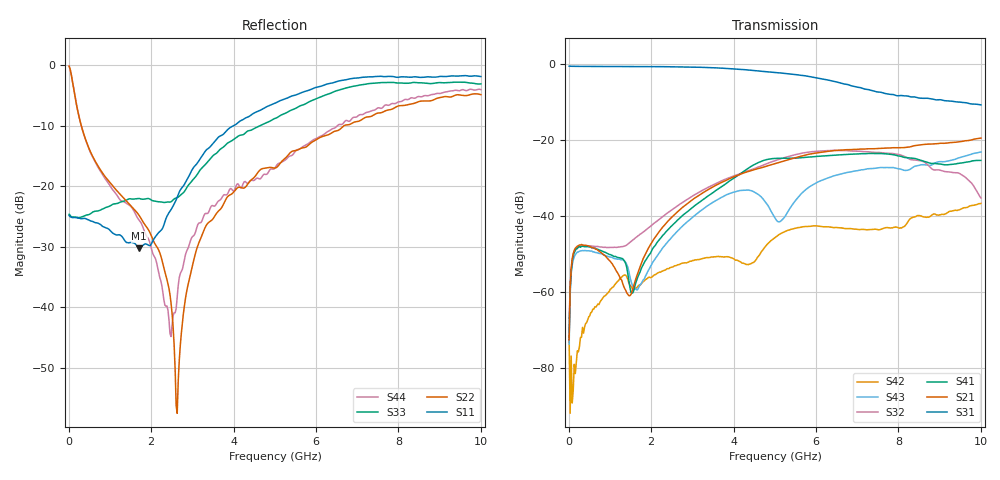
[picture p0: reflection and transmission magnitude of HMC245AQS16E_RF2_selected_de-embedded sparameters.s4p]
! Device:	HMC245AQS16E
! Description:	GaAs MMIC SP3T Non-Reflective Switch
! Package:	LP3E - 16 pin 3x3mm QFN plastic package
! Frequency:	DC -  3.5 GHz
! Ports:
! RFC = Port 1
! RF1 = Port 2
! RF2 = Port 3
! RF3 = Port 4
! State: RF2 Selected
! Supply Voltage:
! Vdd = 5 V
! Control Voltages:
! VA  = 5 V
! VB  = 0 V
! Data:	Data was collected using a calibrated network analyzer with AFR software.
!	Fixtures were calculated using AFR and fixturing was applied to collect
!	this Deembedded  S Parameter data of HMC245AQS16E
! Note:	Analog Devices supplies this data as a sample of measured data at the package pin
!	for this product.  Your particular data for this product may vary.
!	Data was taken at 25 degrees C.
!	Analog Devices reserves the right to change this data at anytime.
# GHz S  dB  R 50
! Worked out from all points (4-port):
!   401 points, 10 MHz to 10 GHz, reference 50 ohm
!   strongest paths, dB at 10 MHz, 2.507 GHz, 5.005 GHz, 7.503 GHz, 10 GHz:
!     S31: -0.6, -0.7, -2.2, -7.4, -10.8
!     S21: -72.6, -40.3, -26.2, -22.2, -19.5
!     S41: -71.9, -42.5, -24.9, -23.6, -25.4
!     S32: -66.9, -38.3, -25.4, -23.3, -35.2
!     S43: -73.7, -45.5, -40.6, -27.3, -23.2
!     S42: -72.6, -53.4, -45.7, -43.6, -36.7
!   lowest |S11| = -30.3 dB at 1.708 GHz (marker M1), VSWR 1.06, Z = 50.8 - j3 ohm
!   |S11| at or under -10 dB: start of sweep to 4.004 GHz
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0.01  -24.85 -1.4  -79.68 119.6  -0.58 -0.4  -71.79 100.1
      -72.58 88.2  -0.18 -5.8  -69.65 130.6  -82.98 -173.8
      -0.57 -0.4  -66.89 106.1  -24.64 -0.9  -83.16 101.8
      -71.86 88.6  -72.59 -80.9  -73.71 63.4  -0.18 -5.8
0.2098  -25.23 -9.2  -48.00 24.9  -0.63 -6.5  -48.37 29.3
        -47.94 24.5  -7.27 -60.3  -48.43 37.4  -76.02 132.0
        -0.63 -6.5  -48.42 37.8  -25.14 -5.9  -49.70 25.7
        -48.54 29.4  -75.45 127.0  -49.51 25.2  -7.24 -60.3
1.7083  -30.25 -73.6  -54.00 169.7  -0.69 -51.9  -55.26 141.3
        -54.07 169.5  -24.82 -63.8  -45.03 90.3  -58.19 71.0
        -0.69 -51.9  -45.05 90.4  -22.02 -38.1  -58.77 146.2
        -55.27 140.5  -58.18 70.4  -58.61 147.5  -25.60 -71.6
2.632375  -21.83 -167.0  -38.97 125.8  -0.74 -81.3  -41.18 121.6
          -38.98 125.8  -57.49 73.7  -37.38 104.5  -52.89 65.2
          -0.74 -81.3  -37.37 104.4  -21.88 -104.5  -44.08 111.2
          -41.17 121.5  -52.91 65.2  -44.00 111.0  -38.29 134.4
3.881125  -10.50 137.3  -30.27 85.2  -1.21 -123.2  -30.93 88.6
          -30.28 85.3  -21.56 104.7  -29.98 85.5  -50.83 42.2
          -1.21 -123.1  -29.97 85.5  -12.78 170.7  -34.20 56.0
          -30.93 88.6  -50.77 41.9  -34.20 56.1  -20.86 102.0
6.728275  -2.42 42.8  -22.56 -0.4  -5.31 146.7  -23.81 -27.0
          -22.56 -0.3  -9.89 49.9  -22.77 11.4  -43.31 13.0
          -5.32 146.8  -22.77 11.4  -3.78 61.9  -28.59 1.4
          -23.82 -27.0  -43.32 13.2  -28.60 1.4  -9.14 46.0
10  -1.89 -27.0  -19.51 -81.4  -10.75 62.4  -25.37 -115.9
    -19.51 -81.4  -4.88 -8.7  -35.24 -59.2  -36.71 13.2
    -10.75 62.4  -35.24 -59.2  -3.11 -16.4  -23.17 -101.8
    -25.37 -115.8  -36.69 13.2  -23.17 -101.7  -4.06 -13.8
